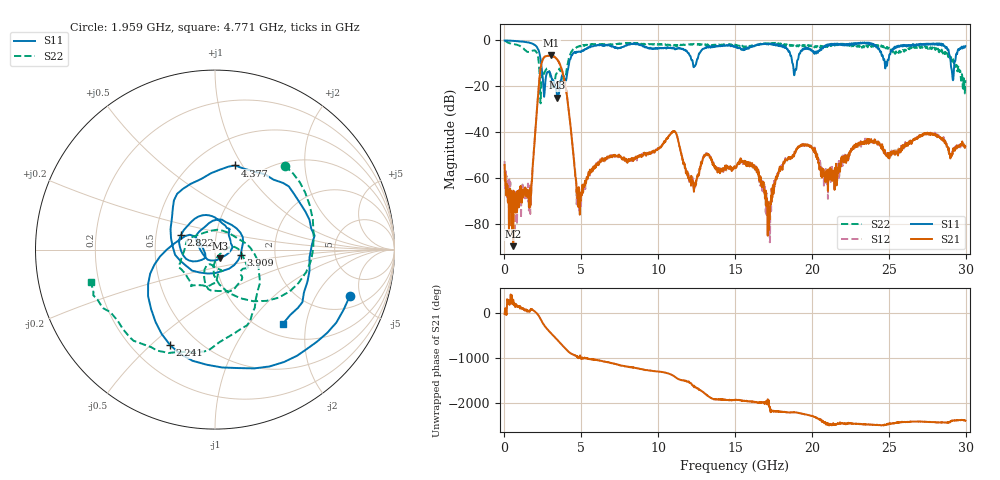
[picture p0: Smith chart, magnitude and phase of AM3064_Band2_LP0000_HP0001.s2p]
# Hz S DB R 50.0
!freq dBS11 angS11 dBS21 angS21 dBS12 angS12 dBS22 angS22
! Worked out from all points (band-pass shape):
!   1600 points, 10 MHz to 29.98 GHz, reference 50 ohm
!   highest |S21| = -6.58 dB at 3.046 GHz (marker M1); lowest = -89.7 dB at 572.3 MHz (marker M2)
!   |S21| within 3 dB of the highest: 2.43 GHz to 3.543 GHz (1.113 GHz wide, 37.3 % of centre)
!   lowest |S11| = -24.9 dB at 3.44 GHz (marker M3), VSWR 1.12, Z = 52.7 - j5.17 ohm
!   |S11| at or under -10 dB: 2.387 GHz to 4.201 GHz (1.815 GHz wide, 55.1 % of centre); 18.73 GHz to 19.02 GHz (287.8 MHz wide, 1.52 % of centre); 29.03 GHz to 29.26 GHz (230.9 MHz wide, 0.792 % of centre)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
!   |S22| runs from -27.4 to -0.2 dB; largest |S21 - S12| = 0.014
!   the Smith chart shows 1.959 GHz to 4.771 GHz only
!   S11 on the Smith chart (normalised r, x): 1.959 GHz: 2.90, -4.03; 2.241 GHz: 0.35, -0.58; 2.822 GHz: 0.68, +0.12; 3.909 GHz: 1.33, -0.08; 4.377 GHz: 0.76, +0.93; 4.771 GHz: 1.22, -1.48
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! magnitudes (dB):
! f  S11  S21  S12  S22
! 10 MHz  0.0  -54.3  -52.6  -0.2
! 572.3 MHz  -0.2  -89.7  -72.7  -1.6
! 1.603 GHz  -1.0  -68.9  -72.7  -5.1
! 1.959 GHz  -2.0  -43.9  -43.7  -4.3
! 2.241 GHz  -4.6  -19.3  -19.2  -10.3
! 2.822 GHz  -13.7  -6.7  -6.6  -12.6
! 3.046 GHz  -15.9  -6.6  -6.6  -19.1
! 3.44 GHz  -24.9  -8.5  -8.4  -13.7
! 3.909 GHz  -16.7  -17.8  -17.7  -19.1
! 4.377 GHz  -6.3  -42.6  -42.4  -4.7
! 4.771 GHz  -5.0  -68.1  -71.1  -2.9
! 5.015 GHz  -4.8  -67.7  -67.5  -2.5
! 10 GHz  -3.4  -47.2  -47.1  -1.7
! 11.09 GHz  -3.9  -39.8  -39.7  -1.9
! 12.31 GHz  -11.7  -64.5  -64.8  -1.6
! 15 GHz  -2.6  -55.2  -55.6  -1.9
! 16.34 GHz  -2.2  -55.3  -54.7  -2.2
! 17.14 GHz  -1.7  -70.4  -74.9  -1.4
! 19.99 GHz  -4.2  -47.0  -47.0  -2.2
! 20.93 GHz  -2.1  -60.1  -59.6  -2.2
! 25 GHz  -8.0  -50.2  -49.3  -3.2
! 29.98 GHz  -2.5  -46.1  -47.2  -17.3
